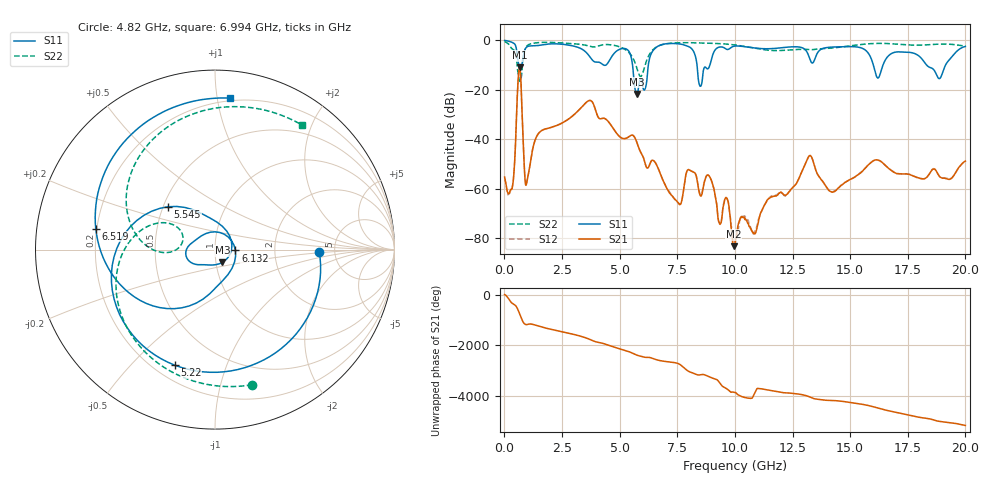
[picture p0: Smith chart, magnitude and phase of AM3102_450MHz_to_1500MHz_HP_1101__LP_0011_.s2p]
!Agilent Technologies,E8364B,MY43040894,A.07.50.67
!Agilent E8364B: A.07.50.67
!Date: Thursday, January 11, 2018 06:37:54
!Correction: S11(Full 2 Port(1,2))
!S21(Full 2 Port(1,2))
!S12(Full 2 Port(1,2))
!S22(Full 2 Port(1,2))
!S2P File: Measurements: S11, S21, S12, S22:
# Hz S  dB  R 50
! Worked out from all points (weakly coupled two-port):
!   1601 points, 10 MHz to 20 GHz, reference 50 ohm
!   highest |S21| = -10.87 dB at 659.7 MHz (marker M1); lowest = -83.2 dB at 9.955 GHz (marker M2)
!   lowest |S11| = -21.7 dB at 5.745 GHz (marker M3), VSWR 1.18, Z = 53.7 - j7.71 ohm
!   |S11| at or under -10 dB: 5.559 GHz to 6.245 GHz (685.3 MHz wide, 11.6 % of centre); 8.357 GHz to 8.916 GHz (559.1 MHz wide, 6.47 % of centre); 18.32 GHz to 19.14 GHz (820 MHz wide, 4.38 % of centre)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
!   |S22| runs from -16.6 to -0.5 dB; largest |S21 - S12| = 0.0016
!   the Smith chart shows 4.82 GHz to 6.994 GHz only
!   S11 on the Smith chart (normalised r, x): 4.82 GHz: 3.77, -0.13; 5.22 GHz: 0.28, -0.67; 5.545 GHz: 0.53, +0.29; 6.132 GHz: 1.26, -0.01; 6.519 GHz: 0.20, +0.08; 6.994 GHz: 0.18, +1.09
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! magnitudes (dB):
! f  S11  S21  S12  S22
! 10 MHz  -0.1  -55.2  -55.8  -0.5
! 347.3 MHz  -0.9  -59.3  -59.0  -3.5
! 659.7 MHz  -11.4  -10.9  -10.9  -16.4
! 972 MHz  -2.7  -57.4  -57.4  -2.3
! 1.484 GHz  -2.1  -37.6  -37.6  -0.9
! 3.346 GHz  -3.5  -27.1  -27.1  -1.7
! 4.82 GHz  -4.7  -37.0  -37.0  -2.2
! 5.22 GHz  -3.3  -39.7  -39.7  -3.6
! 5.545 GHz  -9.0  -38.3  -38.3  -6.7
! 5.745 GHz  -21.7  -41.2  -41.2  -11.1
! 6.132 GHz  -18.9  -50.6  -50.6  -9.2
! 6.519 GHz  -3.4  -49.1  -49.0  -3.2
! 6.682 GHz  -2.3  -51.9  -51.9  -2.3
! 6.994 GHz  -1.4  -58.8  -58.8  -1.4
! 8.868 GHz  -11.1  -54.6  -54.6  -1.2
! 9.955 GHz  -2.4  -83.2  -80.2  -1.8
! 10.01 GHz  -2.3  -82.2  -81.5  -1.9
! 13.34 GHz  -9.1  -47.4  -47.4  -3.8
! 14.22 GHz  -2.7  -61.3  -61.2  -3.1
! 16.68 GHz  -6.1  -51.8  -51.8  -1.3
! 18.86 GHz  -15.5  -54.8  -54.8  -1.5
! 20 GHz  -2.5  -48.8  -48.9  -2.3
